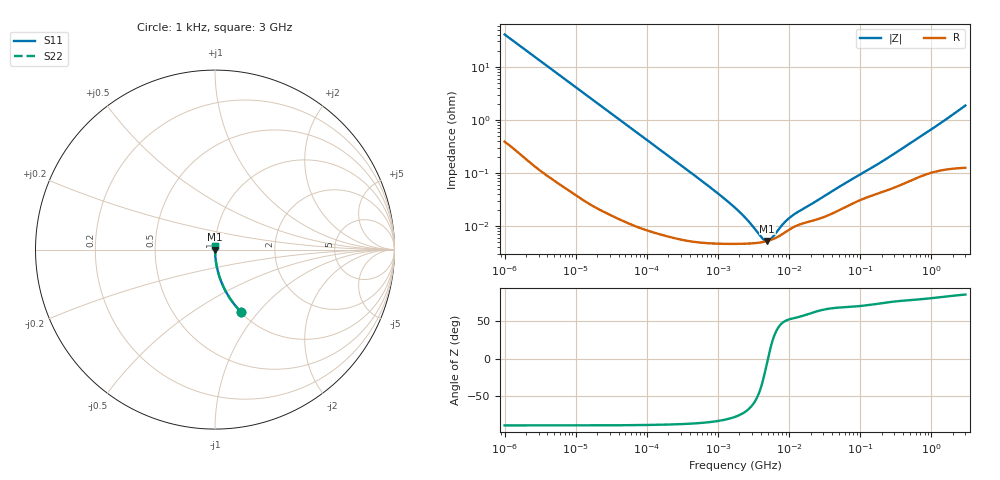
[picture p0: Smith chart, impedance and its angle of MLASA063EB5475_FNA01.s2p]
! MLASA063EB5475_FNA01  S-PARAMETER MODEL  ( Standard Model )
! Model Generated by TAIYO YUDEN Corporation (http://www.ty-top.com)
! Version 1.0
! TAIYO YUDEN Control No. 241206
! Copyright(c) 2024 TAIYO YUDEN CO.,LTD. All Rights Reserved.
! Product Description (link to TY-COMPAS)
! https://ds.yuden.co.jp/TYCOMPAS/or/detail?pn=MLASA063EB5475MFNA01&u=M
! Products Name : Multilayer Ceramic Capacitors
! Characteristics :
!  Capacitance : 4.7 [uF] , Rated Voltage : 4 [V] , TCC : X5R
!  Case Size : 0.6 x 0.3 / 0.024 x 0.012 [mm/inch] , Thickness : 0.3 / 0.012 [mm/inch]
!  (Conditions: Temperature = 25 [degC] , DC Bias Voltage = 0 [V])
! External Node Assignments :
!  1  o---| |---o  2
! GND o---------o GND
! Frequency Range : 1kHz  -  3GHz  [ 401 STEP ]
# MHZ S RI R 50
! Freq[MHz].  S11 Real  S11 Imag  S21 Real  S21 Imag  S12 Real  S12 Imag  S22 Real  S22 Imag
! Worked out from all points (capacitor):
!   401 points, 1 kHz to 3 GHz, reference 50 ohm
!   read as one part in series: C = 3.91 uF near 1.077 kHz
!   lowest |Z| = 5.18 mohm at 4.92 MHz (marker M1)
!   series resonance near 5.032 MHz, so ESL is about 260 pH
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0.001  0.1442 -0.3466  0.8558 0.3466  0.8558 0.3466  0.1442 -0.3466
0.001077  0.1271 -0.3284  0.8729 0.3284  0.8729 0.3284  0.1271 -0.3284
0.001685  0.0572 -0.2278  0.9428 0.2278  0.9428 0.2278  0.0572 -0.2278
0.00306  0.0187 -0.1311  0.9813 0.1311  0.9813 0.1311  0.0187 -0.1311
0.005768  0.00566 -0.0707  0.9943 0.0707  0.9943 0.0707  0.00566 -0.0707
0.01216  0.00146 -0.0338  0.9985 0.0338  0.9985 0.0338  0.00146 -0.0338
0.033275  0.000307 -0.0124  0.9997 0.0124  0.9997 0.0124  0.000307 -0.0124
0.147855  7.81e-05 -0.00283  0.9999 0.00283  0.9999 0.00283  7.81e-05 -0.00283
0.762639  4.72e-05 -0.00054  1 0.00054  1 0.00054  4.72e-05 -0.00054
1.732051  4.58e-05 -0.000215  1 0.000215  1 0.000215  4.58e-05 -0.000215
3.03007  4.69e-05 -8.94e-05  1 8.94e-05  1 8.94e-05  4.69e-05 -8.94e-05
3.264662  4.72e-05 -7.55e-05  1 7.55e-05  1 7.55e-05  4.72e-05 -7.55e-05
4.919932  5.17e-05 -3.8e-06  0.9999 3.8e-06  0.9999 3.8e-06  5.17e-05 -3.8e-06
7.143107  6.36e-05 5.9e-05  0.9999 -5.9e-05  0.9999 -5.9e-05  6.36e-05 5.9e-05
7.696136  6.75e-05 7.13e-05  0.9999 -7.13e-05  0.9999 -7.13e-05  6.75e-05 7.13e-05
11.59828  9.5e-05 0.000133  0.9999 -0.000133  0.9999 -0.000133  9.5e-05 0.000133
21.06097  0.000125 0.000232  0.9999 -0.000232  0.9999 -0.000232  0.000125 0.000232
53.49319  0.000206 0.000533  0.9998 -0.000533  0.9998 -0.000533  0.000206 0.000533
256.0921  0.000489 0.00194  0.9995 -0.00194  0.9995 -0.00194  0.000489 0.00194
1017.49  0.00106 0.00664  0.9989 -0.00664  0.9989 -0.00664  0.00106 0.00664
2784.426  0.00153 0.0172  0.9985 -0.0172  0.9985 -0.0172  0.00153 0.0172
3000  0.00159 0.0185  0.9984 -0.0185  0.9984 -0.0185  0.00159 0.0185
